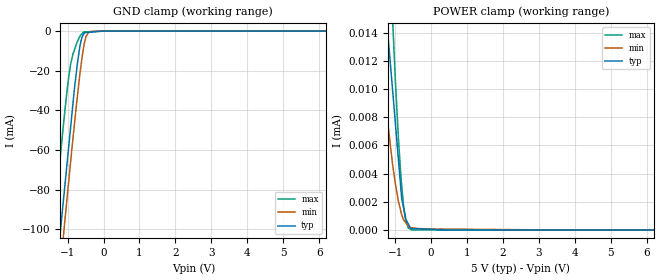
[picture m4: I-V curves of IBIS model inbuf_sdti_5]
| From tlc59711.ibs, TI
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|   inbuf_sdti 5V Model
[Model] inbuf_sdti_5
Model_type   Input
Vinl = 1.5
Vinh = 3.5
|   typ   min   max
|   (nom PVT)   (Fast PVT)   (slow PVT)
C_comp   9.81932E-13   9.72928E-13   9.88328E-13
| Where   nom PVT is  Nominal Process, 5V, 90C
|   Fast PVT is Strong Process, 4.5V, -40C
|   Slow PVT is Weak Process, 5.5V, 150C
|   C_comp - from L-C Tank method, L = 1nH, peak frequency
[Model Spec]
|DVDD   5V   4.5V   5.5V
Vinl   1.5   1.35   1.65
Vinh   3.5   3.15   3.85
|Vinl   0.3 * VREG
|Vinh   0.7 * VREG
| variable   typ   min   max
[Voltage Range]   5   4.5   5.5
|Operating Temperature Range
|   25   85   -40
|Junction Temperature Range
[Temperature Range]   90   150   -40
[Power Clamp Reference]   5   4.5   5.5
[GND Clamp Reference]   0   0   0
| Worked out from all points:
|   GND clamp passes 1 mA (typ) near -0.54 V on its own axis
[GND Clamp]
|   Voltage   I(typ)   I(min)   I(max)
-5V       -858.4mA   -876.5mA   -820.9mA
-1.679V   -193.4mA   -212.4mA   -155mA
-1.238V   -107.4mA   -126.2mA   -69.45mA
-1.135V   -88.47mA   -106.6mA   -50.36mA
-1.053V   -73.52mA   -91.15mA   -36.17mA
-920.1mV  -49.09mA   -66.52mA   -17.12mA
-727.1mV  -16.21mA   -32.73mA   -5.273mA
-653.3mV  -7.124mA   -20.95mA   -2.457mA
-555.3mV  -1.555mA   -8.371mA   -424.7uA
-427.7mV  -624.3uA   -899.3uA   -325.9uA
-164.2mV  -246.6uA   -5.221uA   -121.9uA
9.985V    0A         0A         0A
[POWER Clamp]
|   Voltage   I(typ)   I(min)   I(max)
-5V       81.69uA    57.49uA    104.6uA
-1.483V   25.67uA    15.46uA    44.87uA
-1.248V   15.3uA     8.629uA    26.91uA
-1.16V    12.63uA    6.644uA    20.7uA
-1.062V   9.654uA    4.486uA    14.46uA
-901.6mV  4.787uA    1.954uA    6.196uA
-820.1mV  2.317uA    1.105uA    3.239uA
-769.3mV  1.63uA     729.6nA    1.793uA
-707.4mV  841.2nA    528.5nA    698.2nA
-635.3mV  435.1nA    296.1nA    150.9nA
-530.5mV  106.1nA    155.3nA    0A
9.985V    0A         0A         0A
